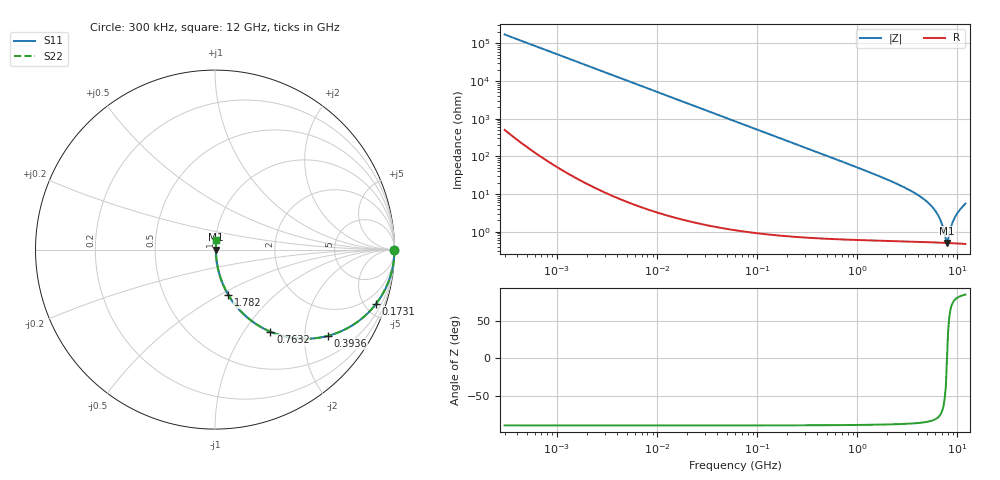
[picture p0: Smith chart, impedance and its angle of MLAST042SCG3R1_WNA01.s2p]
! MLAST042SCG3R1_WNA01  S-PARAMETER MODEL  ( General Type )
! Model Generated by TAIYO YUDEN Corporation (http://www.ty-top.com)
! Version 2.0
! TAIYO YUDEN Control No. 151201
! Copyright(c) 2015 TAIYO YUDEN CO.,LTD. All Rights Reserved.
! Product Description (link to TY-COMPAS)
! https://ds.yuden.co.jp/TYCOMPAS/or/detail?pn=MLAST042SCG3R1BWNA01&u=M
! Products Name : Multilayer Ceramic Capacitors
! Characteristics :
!  Capacitance : 3.1 pF , Rated Voltage : 25V , TCC : CG / C0G
!  Case Size : 0.4 x 0.2 / 0.016 x 0.008 [mm/inch] , Thickness : 0.2 / 0.008 [mm/inch]
!  (Conditions: Temperature = 25 degC , DC Bias Current/Voltage = 0A / 0V)
! External Node Assignments :
!  1  o---| |---o  2
! GND o---------o GND
! Frequency Range : 0.3MHz  -  12000MHz  [ 401 STEP ]
# MHz S RI R 50
! Freq[MHz].  S11 Real  S11 Imag  S21 Real  S21 Imag  S12 Real  S12 Imag  S22 Real  S22 Imag
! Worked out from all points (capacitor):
!   401 points, 300 kHz to 12 GHz, reference 50 ohm
!   read as one part in series: C = 3.1 pF near 316.3 kHz
!   lowest |Z| = 502 mohm at 7.854 GHz (marker M1)
!   series resonance near 7.853 GHz, so ESL is about 130 pH
!   S11 on the Smith chart (normalised r, x): 300 kHz: open; 173.1 MHz: 1.02, -5.93; 393.6 MHz: 1.01, -2.60; 763.2 MHz: 1.01, -1.33; 1.782 GHz: 1.01, -0.55; 12 GHz: 1.01, +0.11
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0.3  1 -0.000584  2.05e-06 0.000584  2.05e-06 0.000584  1 -0.000584
1.769972  1 -0.00345  1.45e-05 0.00345  1.45e-05 0.00345  1 -0.00345
10.44266  0.9996 -0.0203  0.000426 0.0203  0.000426 0.0203  0.9996 -0.0203
60  0.9864 -0.1153  0.0136 0.1153  0.0136 0.1153  0.9864 -0.1153
173.124  0.8972 -0.3024  0.1028 0.3024  0.1028 0.3024  0.8972 -0.3024
353.9943  0.6761 -0.4656  0.3239 0.4656  0.3239 0.4656  0.6761 -0.4656
393.5654  0.6281 -0.4808  0.3719 0.4808  0.3719 0.4808  0.6281 -0.4808
763.2128  0.3091 -0.4575  0.6909 0.4575  0.6909 0.4575  0.3091 -0.4575
1135.593  0.1672 -0.3665  0.8328 0.3665  0.8328 0.3665  0.1672 -0.3665
1781.601  0.0741 -0.2516  0.9259 0.2516  0.9259 0.2516  0.0741 -0.2516
2088.533  0.0544 -0.2148  0.9456 0.2148  0.9456 0.2148  0.0544 -0.2148
3642.919  0.0173 -0.1081  0.9827 0.1081  0.9827 0.1081  0.0173 -0.1081
5278.635  0.00801 -0.0526  0.992 0.0526  0.992 0.0526  0.00801 -0.0526
6524.734  0.00569 -0.0241  0.9943 0.0241  0.9943 0.0241  0.00569 -0.0241
6879.757  0.00537 -0.0172  0.9946 0.0172  0.9946 0.0172  0.00537 -0.0172
7448.838  0.00508 -0.00686  0.9949 0.00686  0.9949 0.00686  0.00508 -0.00686
7854.144  0.005 2.63e-05  0.995 -2.63e-05  0.995 -2.63e-05  0.005 2.63e-05
8281.503  0.00502 0.00708  0.995 -0.00708  0.995 -0.00708  0.00502 0.00708
8966.534  0.00522 0.0173  0.9948 -0.0173  0.9948 -0.0173  0.00522 0.0173
9454.42  0.00545 0.0238  0.9946 -0.0238  0.9946 -0.0238  0.00545 0.0238
10793.46  0.0064 0.04  0.9936 -0.04  0.9936 -0.04  0.0064 0.04
12000  0.00769 0.0544  0.9923 -0.0544  0.9923 -0.0544  0.00769 0.0544
